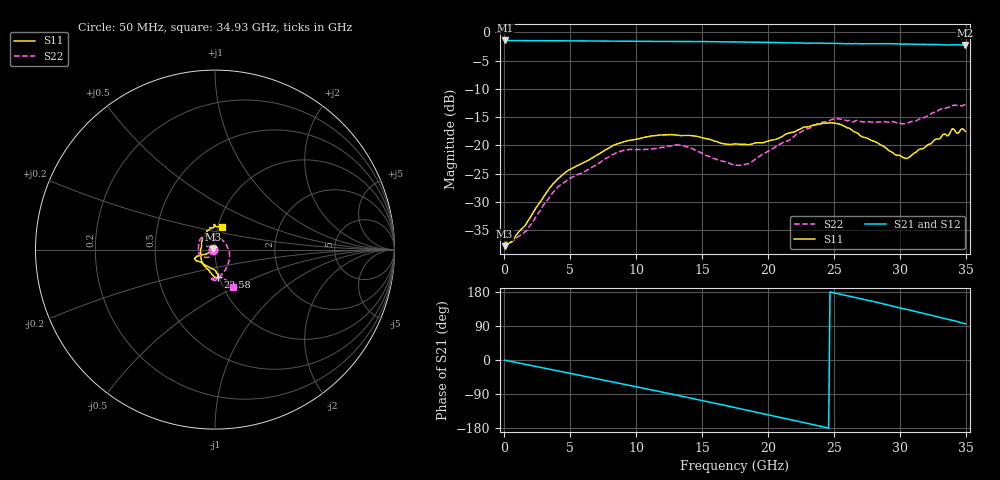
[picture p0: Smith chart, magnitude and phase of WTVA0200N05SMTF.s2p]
! 50 ohm 2-Port S-parameters measured by Modelithics Inc support@modelithics.com  Tampa, FL USA 813-866-6335 (February 2024)
! Smiths Interconnect,  2dB P/N: WTVA0200N05SMTF, Temperature: 75 C
! Board: 10 mil Rogers 4350B, Mounting Pad Dimensions: Length: 15 mils, Width: 25 mils, Gap: 40 mils.
# Hz S RI R 50
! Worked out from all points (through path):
!   352 points, 50 MHz to 34.93 GHz, reference 50 ohm
!   highest |S21| = -1.43 dB at 100 MHz (marker M1); lowest = -2.3 dB at 34.93 GHz (marker M2)
!   group delay of S21, straight-line fit = 20.9 ps
!   lowest |S11| = -37.8 dB at 50 MHz (marker M3), VSWR 1.03, Z = 48.7 + j0.0636 ohm
!   |S11| at or under -10 dB: start of sweep to end of sweep
!   |S22| runs from -37.7 to -12.8 dB; largest |S21 - S12| = 0.01
!   S11 on the Smith chart (normalised r, x): 50 MHz: 0.97, +0.00; 23.58 GHz: 0.99, -0.31; 34.93 GHz: 1.04, +0.27
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5e7  -0.0129 0.000653  0.8478 -0.00467  0.8467 -0.00459  -0.013 -0.000158
1e8  -0.0137 -0.00033  0.8477 -0.0107  0.8469 -0.0109  -0.0139 -0.000658
5.98e8  -0.0139 -0.00276  0.8439 -0.0637  0.8431 -0.0635  -0.0136 -0.00341
1.6925e9  -0.019 -0.00724  0.8258 -0.1756  0.825 -0.1752  -0.0148 -0.00949
3.6825e9  -0.0403 -0.0207  0.7581 -0.3678  0.7568 -0.3683  -0.0232 -0.0302
5.8715e9  -0.0635 -0.0275  0.6305 -0.5548  0.6297 -0.5542  -0.0379 -0.0424
8.8565e9  -0.0994 -0.0362  0.3865 -0.7397  0.3843 -0.7395  -0.0826 -0.0332
1.1742e10  -0.1136 -0.0492  0.1004 -0.825  0.0986 -0.8242  -0.0914 0.0271
1.3533e10  -0.1085 -0.0564  -0.0884 -0.8258  -0.0901 -0.8247  -0.0723 0.0687
1.7513e10  -0.0583 -0.0852  -0.4828 -0.6677  -0.4829 -0.6664  0.0441 0.0503
1.8508e10  -0.0383 -0.0944  -0.5632 -0.5949  -0.5634 -0.5936  0.0662 0.0195
2.05975e10  -0.00193 -0.1133  -0.6998 -0.4137  -0.6994 -0.4125  0.0788 -0.0581
2.33835e10  0.017 -0.1501  -0.7916 -0.1349  -0.7906 -0.1349  0.0308 -0.1448
2.35825e10  0.0171 -0.1519  -0.7951 -0.1141  -0.7943 -0.112  0.0282 -0.1501
2.5473e10  -0.00129 -0.1532  -0.7915 0.0939  -0.7905 0.0941  -0.00848 -0.171
2.91545e10  -0.0777 -0.0444  -0.646 0.462  -0.6405 0.4674  0.00526 -0.1601
3.0448e10  -0.0752 0.0148  -0.5465 0.5679  -0.5403 0.5723  0.0309 -0.1538
3.3234e10  -0.0264 0.1221  -0.2709 0.7294  -0.2662 0.73  0.0794 -0.1973
3.3632e10  -0.0102 0.1215  -0.2292 0.7382  -0.2225 0.7392  0.0839 -0.2006
3.39305e10  -0.00215 0.1403  -0.1972 0.7494  -0.1913 0.7499  0.0907 -0.2045
3.43285e10  0.0127 0.1272  -0.1486 0.7631  -0.1441 0.7629  0.0897 -0.2072
3.49255e10  0.0382 0.1273  -0.0757 0.7676  -0.075 0.7662  0.099 -0.2078
